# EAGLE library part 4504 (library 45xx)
TTL or CMOS to CMOS hex LEVEL SHIFTER
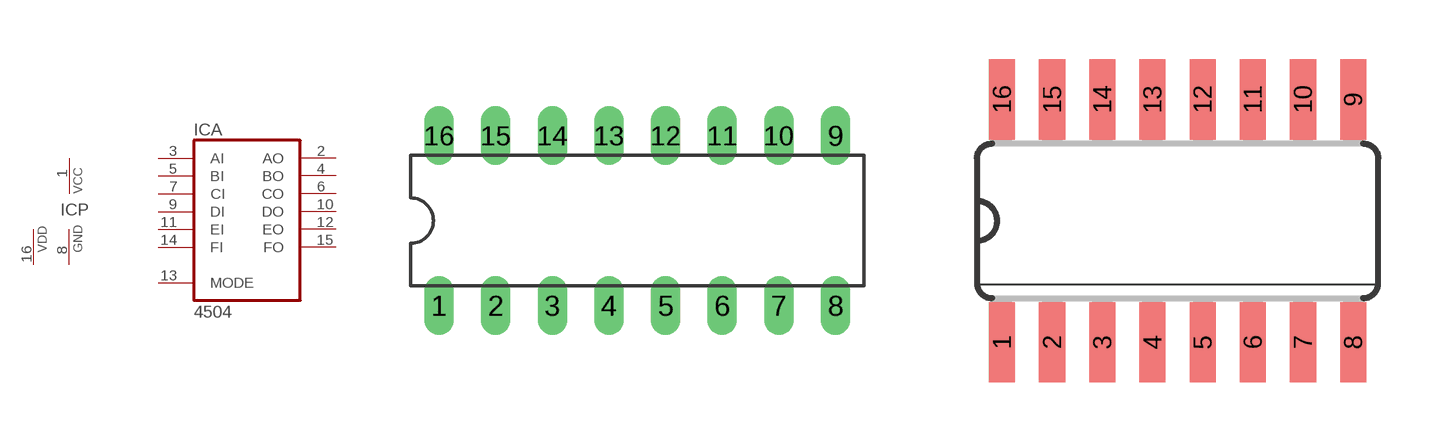
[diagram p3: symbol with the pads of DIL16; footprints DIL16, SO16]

Designator prefix IC; gates A=4504 P=PWR+VCC

## 4504N  [DIL16]
1  P:VCC  pwr
2  A:AO  out
3  A:AI  in
4  A:BO  out
5  A:BI  in
6  A:CO  out
7  A:CI  in
8  P:GND  pwr
9  A:DI  in
10  A:DO  out
11  A:EI  in
12  A:EO  out
13  A:MODE  in
14  A:FI  in
15  A:FO  out
16  P:VDD  pwr

## 4504D  [SO16]
Pads as for DIL16

## Footprint DIL16 (pad centres in mm)
Dual In Line Package
drill 0.813 long: 1 -8.89,-3.81; 2 -6.35,-3.81; 3 -3.81,-3.81; 4 -1.27,-3.81; 5 1.27,-3.81; 6 3.81,-3.81; 7 6.35,-3.81; 8 8.89,-3.81; 9 8.89,3.81; 10 6.35,3.81; 11 3.81,3.81; 12 1.27,3.81; 13 -1.27,3.81; 14 -3.81,3.81; 15 -6.35,3.81; 16 -8.89,3.81

## Footprint SO16 (pad centres in mm)
Small Outline package 150 mil
smd 0.66 x 2.032: 1 -4.445,-3.073; 2 -3.175,-3.073; 3 -1.905,-3.073; 4 -0.635,-3.073; 5 0.635,-3.073; 6 1.905,-3.073; 7 3.175,-3.073; 8 4.445,-3.073; 9 4.445,3.073; 10 3.175,3.073; 11 1.905,3.073; 12 0.635,3.073; 13 -0.635,3.073; 14 -1.905,3.073; 15 -3.175,3.073; 16 -4.445,3.073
